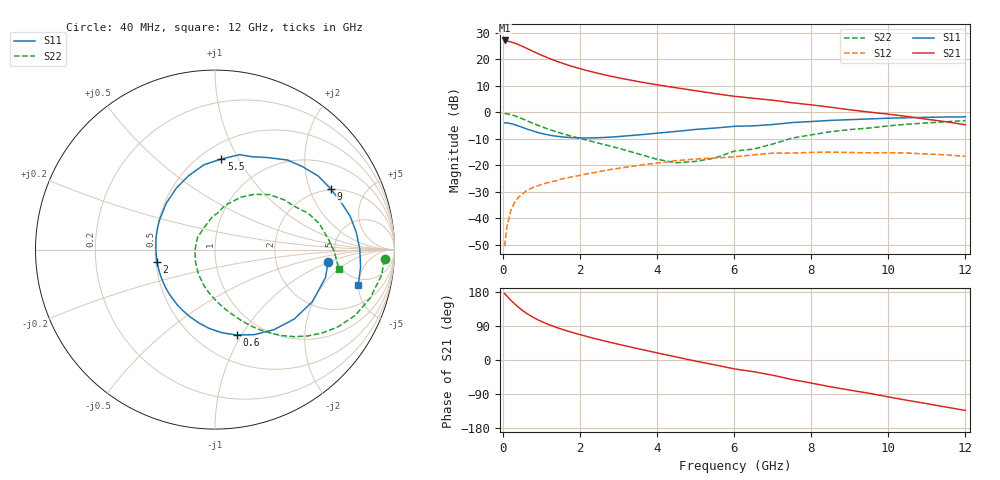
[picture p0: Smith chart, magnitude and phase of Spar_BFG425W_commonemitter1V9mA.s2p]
! Filename: 19bfg425.001
! BFG425W Field C1
! V1=8.506E-001V,V2=1.000E+000V, I1=1.302E-004A, I2=9.000E-003A
# GHz  S  MA  R 50
!  S11  S21  S12  S22
!Freq(GHz)  Mag  Ang  Mag  Ang  Mag  Ang  Mag  Ang
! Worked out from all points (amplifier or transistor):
!   44 points, 40 MHz to 12 GHz, reference 50 ohm
!   highest |S21| = 27.1 dB at 40 MHz (marker M1)
!   |S21| within 3 dB of that: start of sweep to 616.2 MHz
!   unconditionally stable (mu >= 1): 1.876 GHz to end of sweep
!   at 700 MHz: K = 0.52, MSG = 26.2 dB, |S12| = -28.9 dB
!   at 2.4 GHz: K = 1.11, MAG = 16.7 dB, |S12| = -22.6 dB
!   at 12 GHz: K = 1.40, MAG = 2.2 dB, |S12| = -16.6 dB
!   S11 on the Smith chart (normalised r, x): 40 MHz: 4.23, -0.98; 600 MHz: 0.76, -0.95; 2 GHz: 0.51, -0.08; 5.5 GHz: 0.63, +0.85; 9 GHz: 1.96, +2.82; 12 GHz: 4.09, -4.95
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0.04  0.634 -6.3  22.69 175.1  0.003 80.2  0.946 -3.3
0.1  0.635 -14.3  22.18 168.7  0.007 82.9  0.939 -8.6
0.2  0.615 -28.3  21.32 157.8  0.014 75.6  0.906 -17.3
0.3  0.587 -41.2  20.25 148.3  0.02 69.6  0.863 -25.1
0.4  0.554 -53.6  18.95 139.2  0.025 64.5  0.81 -32.1
0.5  0.522 -65.2  17.62 130.9  0.029 60.1  0.756 -38.0
0.6  0.491 -75.7  16.27 123.8  0.033 56.5  0.704 -43.2
0.8  0.44 -94.3  13.9 111.6  0.039 50.9  0.611 -51.7
0.9  0.418 -102.5  12.89 106.3  0.041 49.0  0.571 -55.3
1  0.4 -110.2  11.96 101.5  0.044 47.4  0.536 -58.4
1.2  0.373 -124.1  10.41 93.0  0.048 44.7  0.476 -64.1
1.6  0.341 -148.1  8.164 78.8  0.057 40.9  0.386 -73.5
2  0.33 -167.9  6.655 66.9  0.065 37.6  0.323 -82.3
2.2  0.329 -176.8  6.082 61.4  0.07 35.8  0.296 -86.7
3  0.35 152.4  4.475 41.4  0.088 27.6  0.21 -106.9
4.5  0.438 109.4  2.902 7.9  0.123 7.8  0.112 -177.6
5.5  0.506 86.0  2.257 -12.9  0.138 -7.0  0.138 115.5
6.5  0.557 68.3  1.843 -30.8  0.158 -18.7  0.203 86.1
8.5  0.706 35.5  1.251 -70.7  0.178 -54.2  0.431 45.3
9  0.729 27.6  1.118 -79.4  0.175 -62.0  0.474 35.9
10.5  0.793 7.0  0.835 -106.6  0.171 -87.6  0.599 14.0
12  0.822 -13.8  0.583 -133.2  0.148 -115.9  0.697 -8.7
